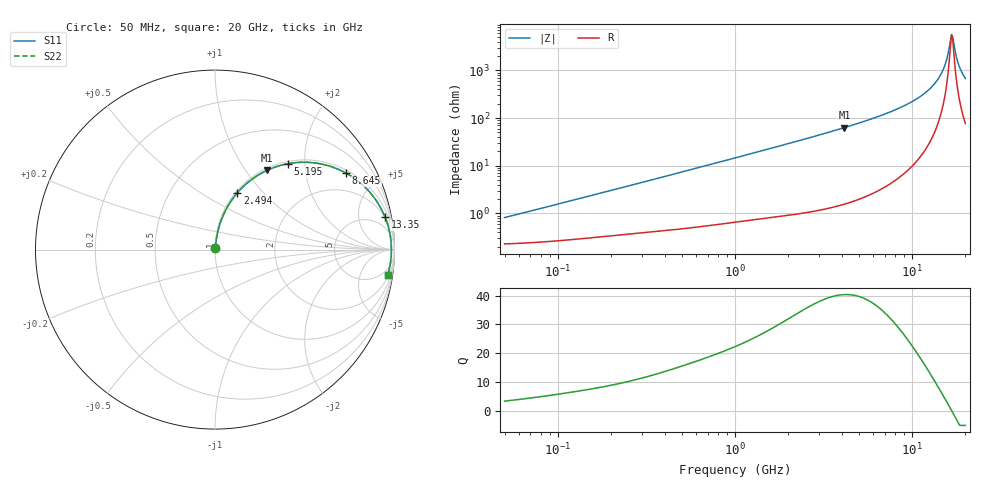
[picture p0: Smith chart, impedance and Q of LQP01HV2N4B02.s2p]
!Murata Part Number: LQP01HV2N4B02
!These Parameters are Measured in Series Mode Connection
!  o--[Z]--o
!Port1  Port2
!  o-------o
!Freq. Start=50[MHz] Stop=20[GHz], 401[Steps]
# Hz S RI R 50
!Freq.(Hz) S11(Real) S11(Imag) S21(Real) S21(Imag) S12(Real) S12(Imag) S22(Real) S22(Imag)
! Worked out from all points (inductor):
!   401 points, 50 MHz to 20 GHz, reference 50 ohm
!   read as one part in series: L = 2.49 nH near 51.52 MHz
!   highest Q = 40.3 at 4.149 GHz (marker M1), where L = 2.42 nH
!   self-resonance near 16.71 GHz
!   S11 on the Smith chart (normalised r, x): 50 MHz: 1.00, +0.02; 2.494 GHz: 1.02, +0.73; 5.195 GHz: 1.04, +1.64; 8.645 GHz: 1.12, +3.35; 13.35 GHz: 2, +10; 20 GHz: 3, -13
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5e7  0.00235 0.00782  0.9977 -0.00782  0.9977 -0.00782  0.00235 0.00782
1.364002e8  0.00338 0.0208  0.9966 -0.0208  0.9966 -0.0208  0.00338 0.0208
3.721004e8  0.0072 0.0546  0.9928 -0.0546  0.9928 -0.0546  0.0072 0.0546
1e9  0.0268 0.1407  0.9732 -0.1407  0.9732 -0.1407  0.0268 0.1407
2.493527e9  0.1244 0.3163  0.8756 -0.3163  0.8756 -0.3163  0.1244 0.3163
2.728004e9  0.1451 0.3389  0.8549 -0.3389  0.8549 -0.3389  0.1451 0.3389
4.149438e9  0.2894 0.4413  0.7106 -0.4413  0.7106 -0.4413  0.2894 0.4413
5.194772e9  0.4042 0.4782  0.5958 -0.4782  0.5958 -0.4782  0.4042 0.4782
7.442007e9  0.6316 0.4672  0.3684 -0.4672  0.3684 -0.4672  0.6316 0.4672
8.644534e9  0.7304 0.4261  0.2696 -0.4261  0.2696 -0.4261  0.7304 0.4261
1.115139e10  0.8771 0.3021  0.1229 -0.3021  0.1229 -0.3021  0.8771 0.3021
1.334722e10  0.9481 0.1796  0.0519 -0.1796  0.0519 -0.1796  0.9481 0.1796
1.417136e10  0.9637 0.1342  0.0363 -0.1342  0.0363 -0.1342  0.9637 0.1342
1.504638e10  0.9748 0.0873  0.0252 -0.0873  0.0252 -0.0873  0.9748 0.0873
1.573793e10  0.98 0.0514  0.02 -0.0514  0.02 -0.0514  0.98 0.0514
1.646126e10  0.9826 0.0152  0.0174 -0.0152  0.0174 -0.0152  0.9826 0.0152
1.670968e10  0.9829 0.00309  0.0171 -0.00309  0.0171 -0.00309  0.9829 0.00309
1.721783e10  0.9825 -0.0211  0.0175 0.0211  0.0175 0.0211  0.9825 -0.0211
1.800918e10  0.9798 -0.0573  0.0202 0.0573  0.0202 0.0573  0.9798 -0.0573
1.855685e10  0.9764 -0.0813  0.0236 0.0813  0.0236 0.0813  0.9764 -0.0813
1.940974e10  0.9692 -0.1168  0.0308 0.1168  0.0308 0.1168  0.9692 -0.1168
2e10  0.963 -0.1401  0.037 0.1401  0.037 0.1401  0.963 -0.1401
